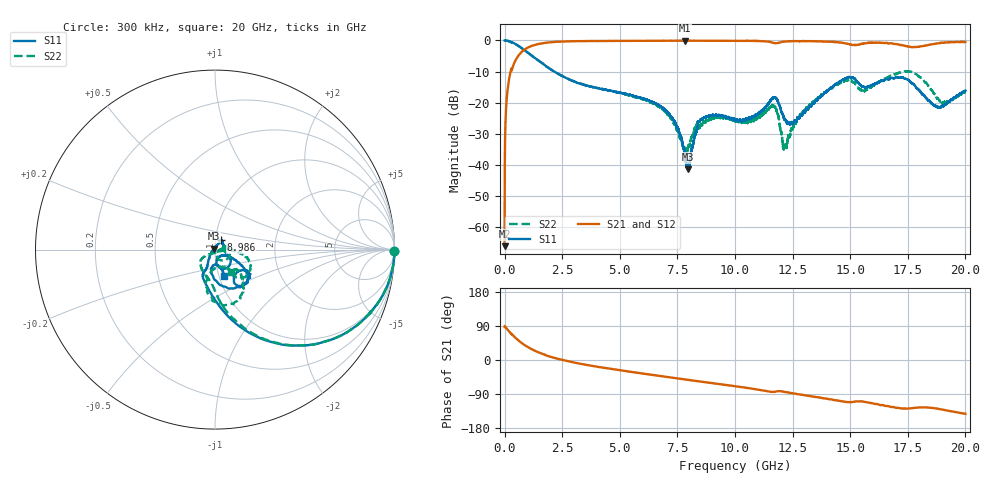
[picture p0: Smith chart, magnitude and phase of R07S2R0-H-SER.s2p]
!{R07S2R0}
!Johanson Technology Inc.
!www.johansontechnology.com
!Test Board Conditions:
!Substrate Type  RO4350B
!Substrate Thickness  10 mil
!Substrate Dk  3.66
!TL Type: GCPW
!TL Trace Width  21 mil
!TL Gap  20 mil
!Electrode orientation  Horizontal
!DUT TOPOLOGY	SERIES
!Mounting Pad LxW  16x21 mil
! Created Sat Feb  6 11:26:31 2021
# hz S ma R 50
! 2 Port Network Data from SP1.SP block
! freq  magS11  angS11  magS21  angS21  magS12  angS12  magS22  angS22
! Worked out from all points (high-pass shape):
!   20001 points, 300 kHz to 20 GHz, reference 50 ohm
!   highest |S21| = -0.06 dB at 7.828 GHz (marker M1); lowest = -66.2 dB at 300 kHz (marker M2)
!   |S21| within 3 dB of the highest: 845.5 MHz to end of sweep
!   lowest |S11| = -41.5 dB at 7.957 GHz (marker M3), VSWR 1.02, Z = 49.3 + j0.526 ohm
!   |S11| at or under -10 dB: 2.16 GHz to end of sweep
!   |S22| runs from -36.4 to 0.0 dB; largest |S21 - S12| = 0.014
!   S11 on the Smith chart (normalised r, x): 300 kHz: open; 8.986 GHz: 1.06, +0.11; 20 GHz: 1.06, -0.32
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300000  0.998 -0.4  0.0004907 86.7  0.0003531 97.6  1 -0.3
1.013e8  0.9908 -7.9  0.1275 82.4  0.1276 82.4  0.9905 -7.8
1.313e8  0.9856 -10.3  0.1647 79.9  0.1645 80.0  0.9857 -10.3
4.843e8  0.8697 -31.7  0.4867 57.9  0.4867 57.9  0.8707 -31.8
1.5373e9  0.4551 -71.7  0.886 18.7  0.8871 18.6  0.4573 -70.1
3.3343e9  0.1984 -105.0  0.9756 -10.5  0.9759 -10.5  0.2002 -94.0
6.6673e9  0.09132 -116.5  0.9889 -41.4  0.9893 -41.5  0.08715 -145.5
7.4413e9  0.04374 -129.7  0.9909 -47.9  0.9915 -48.0  0.04027 -137.5
7.8283e9  0.01438 -163.8  0.9934 -51.3  0.9917 -51.3  0.01772 -86.4
7.9573e9  0.008449 140.9  0.9905 -52.4  0.9906 -52.4  0.0189 -50.3
8.4543e9  0.04943 57.6  0.9902 -56.5  0.9895 -56.6  0.03922 2.9
8.9863e9  0.06184 58.8  0.9882 -60.8  0.988 -60.9  0.05483 -9.0
1.00003e10  0.0536 29.7  0.9864 -69.2  0.9874 -69.3  0.05045 -1.9
1.16863e10  0.1218 -52.2  0.9122 -84.0  0.9109 -84.1  0.08823 -32.6
1.21693e10  0.05283 -74.3  0.9613 -84.2  0.9597 -84.3  0.02101 -31.8
1.33343e10  0.09221 -25.3  0.9722 -95.9  0.9727 -96.0  0.09807 -3.7
1.48733e10  0.252 -44.5  0.8869 -110.8  0.8882 -110.9  0.2279 -33.3
1.55783e10  0.1808 -51.5  0.8932 -110.1  0.8953 -110.0  0.1561 -46.6
1.66673e10  0.237 -36.1  0.8949 -121.9  0.899 -122.5  0.2577 -52.3
1.78213e10  0.1861 -85.1  0.7853 -126.0  0.7842 -125.9  0.2924 -89.6
1.88403e10  0.08472 -88.7  0.9033 -129.0  0.9031 -129.1  0.113 -95.1
2e10  0.1562 -70.6  0.9462 -142.1  0.9418 -142.1  0.1521 -54.4
